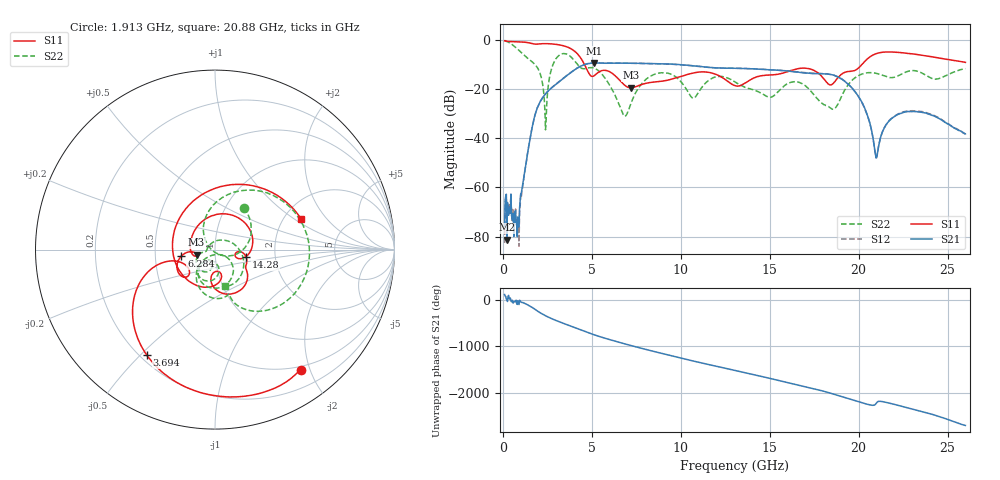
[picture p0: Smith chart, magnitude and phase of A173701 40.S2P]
!  2-Port S-parameters saved by WinCal
! VAR MeasName=S-Parameters (CALIBRATED_DATA) read from VNA (N5245A)
! VAR MeasDate=2017-6-7 10:31:03
! VAR NAME=A173701 40
! VAR FILENAME=A173701 40.S2P
! VAR DATE=2017-6-7 10:31:03
! VAR PHYS_PORTS=1,2
# Hz S DB R 50
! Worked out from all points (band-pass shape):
!   801 points, 100 MHz to 26 GHz, reference 50 ohm
!   highest |S21| = -9.37 dB at 5.151 GHz (marker M1); lowest = -81.2 dB at 229.5 MHz (marker M2)
!   |S21| within 3 dB of the highest: 3.995 GHz to 15.52 GHz (11.53 GHz wide, 118 % of centre)
!   lowest |S11| = -19.5 dB at 7.19 GHz (marker M3), VSWR 1.24, Z = 40.6 - j2.33 ohm
!   |S11| at or under -10 dB: 4.589 GHz to 20.18 GHz (15.59 GHz wide, 126 % of centre)
!   |S22| runs from -36.6 to -0.2 dB; largest |S21 - S12| = 0.0054
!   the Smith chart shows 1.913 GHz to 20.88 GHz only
!   S11 on the Smith chart (normalised r, x): 1.913 GHz: 0.45, -1.85; 3.694 GHz: 0.23, -0.52; 6.284 GHz: 0.68, -0.05; 14.28 GHz: 1.41, -0.12; 20.88 GHz: 2.47, +1.14
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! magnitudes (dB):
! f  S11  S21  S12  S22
! 100 MHz  -0.3  -75.9  -82.5  -0.2
! 229.5 MHz  -0.6  -81.2  -76.6  -0.6
! 877 MHz  -0.8  -75.9  -75.9  -4.0
! 1.913 GHz  -1.7  -28.1  -28.1  -11.0
! 2.399 GHz  -1.5  -22.0  -21.9  -36.6
! 2.884 GHz  -1.7  -18.6  -18.6  -9.0
! 3.694 GHz  -3.1  -14.0  -13.9  -6.2
! 4.438 GHz  -8.0  -10.4  -10.4  -11.6
! 5.151 GHz  -14.5  -9.4  -9.4  -11.6
! 6.284 GHz  -14.4  -9.5  -9.4  -22.1
! 7.19 GHz  -19.5  -9.5  -9.5  -26.0
! 8.744 GHz  -16.9  -9.7  -9.7  -13.5
! 10.69 GHz  -13.5  -10.5  -10.6  -23.7
! 13.05 GHz  -18.6  -11.5  -11.5  -17.1
! 14.28 GHz  -15.0  -11.9  -11.8  -20.8
! 17.39 GHz  -12.1  -13.7  -13.5  -21.4
! 18.59 GHz  -17.6  -14.3  -14.3  -28.2
! 19.69 GHz  -12.6  -20.0  -20.1  -16.0
! 20.88 GHz  -5.9  -43.6  -43.7  -13.4
! 21.69 GHz  -4.9  -33.1  -32.9  -15.2
! 23.54 GHz  -6.2  -29.5  -29.1  -13.4
! 26 GHz  -9.1  -38.2  -38.2  -11.7
